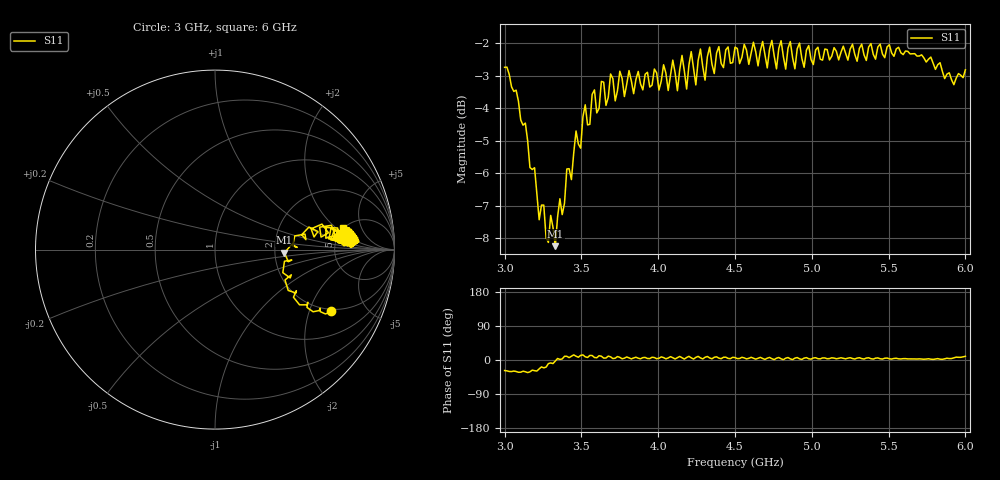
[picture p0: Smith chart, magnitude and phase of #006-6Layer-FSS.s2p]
!  05/08/2025  16:59:45
! Ref Plane: 0.000 mm
# MHZ S MA R  50
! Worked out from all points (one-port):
!   201 points, 3 GHz to 6 GHz, reference 50 ohm
!   lowest |S11| = -8.2 dB at 3.33 GHz (marker M1), VSWR 2.26, Z = 113 - j4.54 ohm
!   |S11| at or under -10 dB: nowhere
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3000  0.7295 -27.8
3150  0.5626 -33.1
3330  0.3872 -2.5
3375  0.433 2.8
3510  0.6125 13.4
3750  0.7195 6.9
4065  0.672 5.4
4095  0.7483 6.0
4125  0.6715 6.1
4155  0.7608 5.8
4185  0.6755 6.5
4215  0.7712 5.7
4245  0.6855 6.9
4275  0.7783 5.5
4305  0.697 7.2
4335  0.7836 5.4
4365  0.7136 7.2
4500  0.7833 6.5
4695  0.7627 1.6
4725  0.7783 6.8
4755  0.7602 1.1
4785  0.7799 6.6
4815  0.7575 0.9
4845  0.7803 6.5
4875  0.7547 1.1
5250  0.7784 6.0
5625  0.7719 2.9
6000  0.7231 9.7
